PROGRAM MAIN
VAR
	aPoints : ARRAY [1..2,1..100] OF ST_Point;
	
	bInit : BOOL := TRUE;
	nCounter: INT;
	nValue1 : INT := 1;
	nValue2 : INT := -1;
END_VAR

IF bInit THEN
	FOR nCounter := 1 TO 100 DO
		aPoints[1, nCounter].x := nCounter;
		aPoints[2, nCounter].x := nCounter;
		aPoints[2, nCounter].y := 100;
	END_FOR
	
	bInit := FALSE;
END_IF

// graph 1
FOR nCounter := 100 TO 2 BY -1 DO
	aPoints[1, nCounter].y := aPoints[1, nCounter - 1].y;
END_FOR

aPoints[1, 1].y := aPoints[1, 1].y + nValue1;

IF aPoints[1, 1].y = 100 THEN
	nValue1 := -1;
ELSIF aPoints[1, 1].y = 1 THEN
	nValue1 := 1;
END_IF 

// graph 2
FOR nCounter := 100 TO 2 BY -1 DO
	aPoints[2, nCounter].y := aPoints[2, nCounter - 1].y;
END_FOR

aPoints[2, 1].y := aPoints[2, 1].y + nValue2;

IF aPoints[2, 1].y = 100 THEN
	nValue2 := -1;
ELSIF aPoints[2, 1].y = 1 THEN
	nValue2 := 1;
END_IF

END_PROGRAM
